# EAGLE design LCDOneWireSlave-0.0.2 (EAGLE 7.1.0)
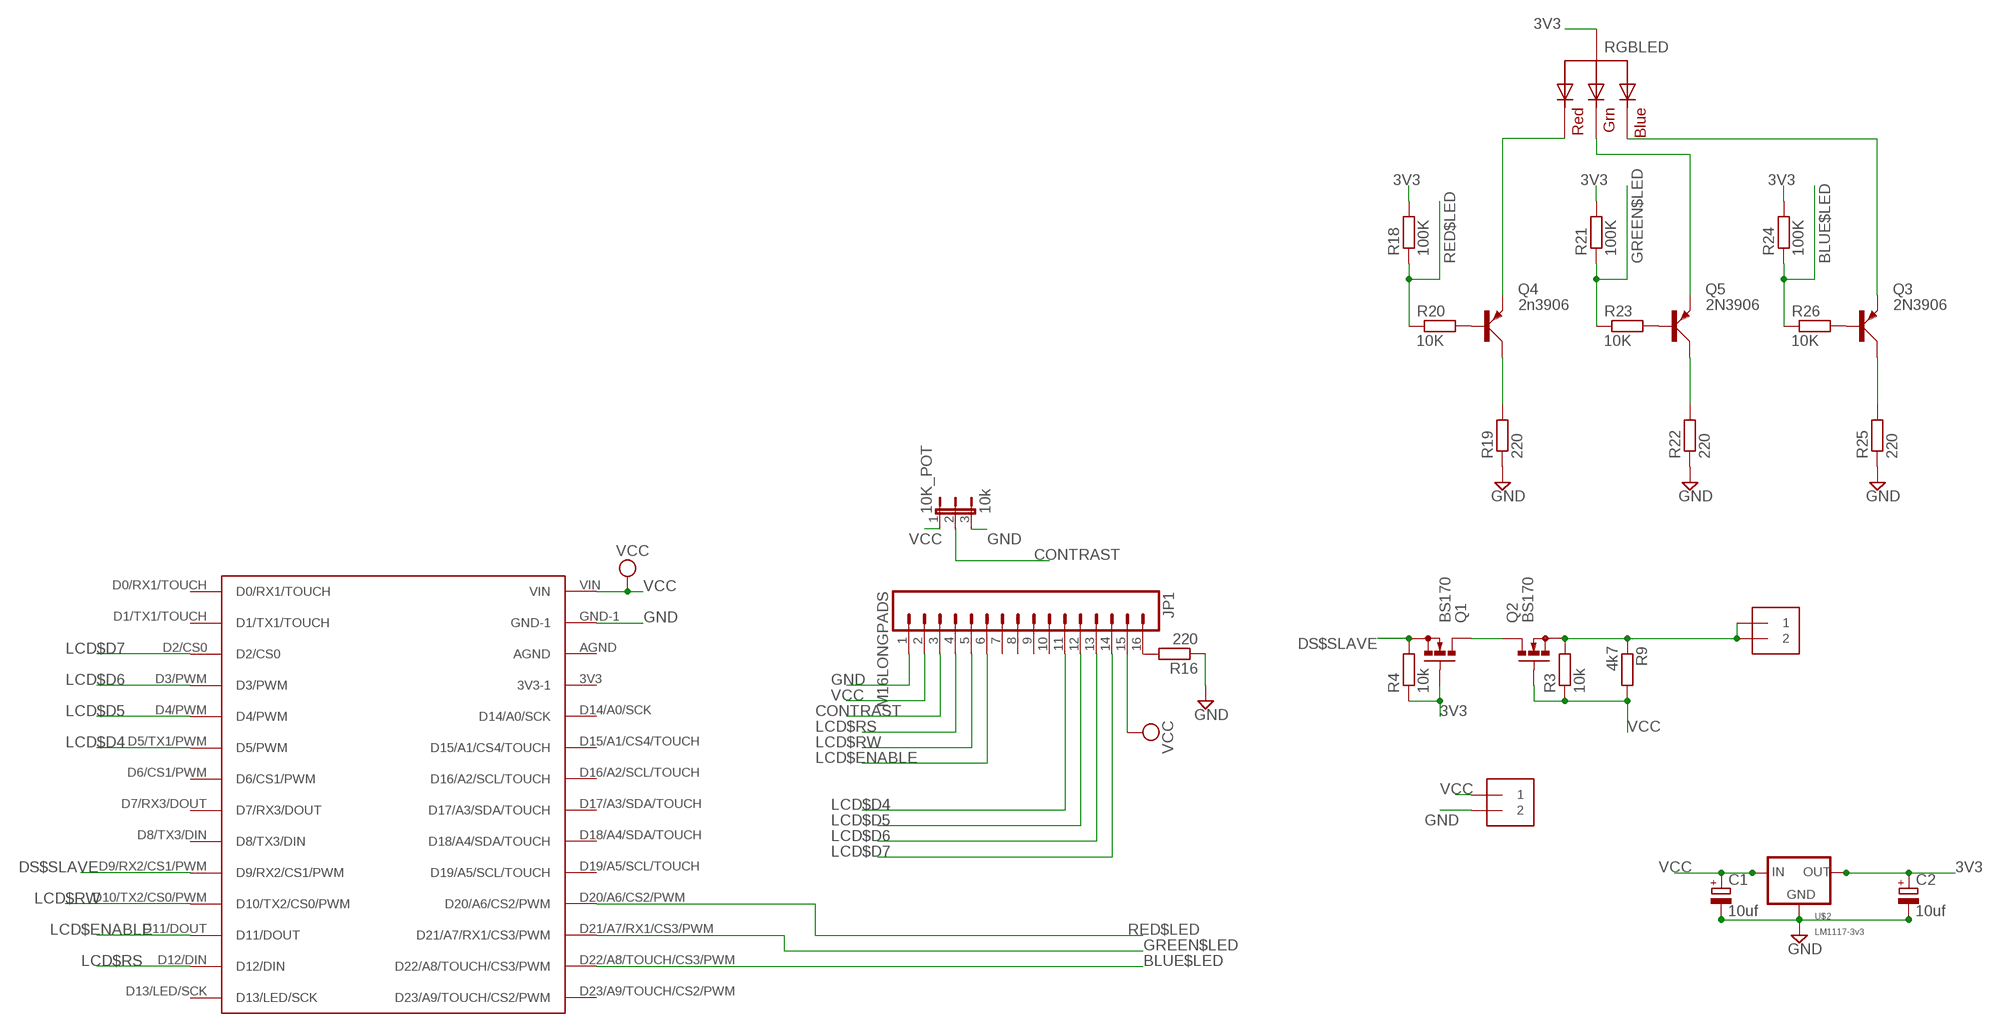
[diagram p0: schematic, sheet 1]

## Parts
10K_POT  10k  JP2E  [JP2]
C1  10uf  CPOL-EUE5-4  [E5-4]
C2  10uf  CPOL-EUE5-4  [E5-4]
DATA  1X2-3.5MM  [1X2-3.5MM]
JP1  M16LONGPADS  [1X16_LONGPADS]
POWER  1X2-3.5MM  [1X2-3.5MM]
Q1  BS170  [SOT54E]
Q2  BS170  [SOT54E]
Q3  2N3906  [TO92D]
Q4  2n3906  2N3906  [TO92D]
Q5  2N3906  [TO92D]
R3  10k  R-EU_0207/10  [0207/10]
R4  10k  R-EU_0207/10  [0207/10]
R9  4k7  R-EU_0207/10  [0207/10]
R16  220  R-EU_0207/10  [0207/10]
R18  100K  R-EU_0207/10  [0207/10]
R19  220  R-EU_0207/10  [0207/10]
R20  10K  R-EU_0207/10  [0207/10]
R21  100K  R-EU_0207/10  [0207/10]
R22  220  R-EU_0207/10  [0207/10]
R23  10K  R-EU_0207/10  [0207/10]
R24  100K  R-EU_0207/10  [0207/10]
R25  220  R-EU_0207/10  [0207/10]
R26  10K  R-EU_0207/10  [0207/10]
RGBLED  RGBLED_CA-5MM  [LED5MMRGB]
U$1  TEENSY30-FULL  [TEENSY30-FULL]
U$2  LM1117-3v3  V_REG_LD1117VXX  [78XXL]

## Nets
3V3 [3v3]: C2.+ Q1.G R4.1 R18.2 R21.2 R24.2 RGBLED.2(VCC) U$2.GND(OUT)
BLUE$LED: R24.1 R26.1 U$1.D22/A8/TOUCH/CS3/PWM
CONTRAST: 10K_POT.2 JP1.3
DS$SLAVE: Q1.S R4.2 U$1.D9/RX2/CS1/PWM
GND [GND]: 10K_POT.3 C1.- C2.- JP1.1 POWER.2 R16.1 R19.1 R22.1 R25.1 U$1.GND-1 U$2.IN(GND)
GREEN$LED: R21.1 R23.1 U$1.D21/A7/RX1/CS3/PWM
LCD$D4: JP1.11 U$1.D5/TX1/PWM(D5/PWM)
LCD$D5: JP1.12 U$1.D4/PWM
LCD$D6: JP1.13 U$1.D3/PWM
LCD$D7: JP1.14 U$1.D2/CS0
LCD$ENABLE: JP1.6 U$1.D11/DOUT
LCD$RS: JP1.4 U$1.D12/DIN
LCD$RW: JP1.5 U$1.D10/TX2/CS0/PWM
N$1: DATA.1 DATA.2 Q2.S R3.2 R9.1
N$2: Q4.E RGBLED.1(RED)
N$3: Q5.E RGBLED.3(GREEN)
N$4: Q3.E RGBLED.4(BLUE)
N$5: Q4.C R19.2
N$6: JP1.16 R16.2
N$7: Q5.C R22.2
N$8: Q3.C R25.2
N$10: Q4.B R20.2
N$15: Q5.B R23.2
N$22: Q3.B R26.2
N$26: Q1.D Q2.D
RED$LED: R18.1 R20.1 U$1.D20/A6/CS2/PWM
VCC [VCC]: 10K_POT.1 C1.+ JP1.2 JP1.15 POWER.1 Q2.G R3.1 R9.2 U$1.VIN U$2.OUT(IN)
Unconnected: JP1.7 JP1.8 JP1.9 JP1.10 U$1.3V3(3V3-1) U$1.AGND U$1.D0/RX1/TOUCH U$1.D1/TX1/TOUCH U$1.D6/CS1/PWM U$1.D7/RX3/DOUT U$1.D8/TX3/DIN U$1.D13/LED/SCK U$1.D14/A0/SCK U$1.D15/A1/CS4/TOUCH U$1.D16/A2/SCL/TOUCH U$1.D17/A3/SDA/TOUCH U$1.D18/A4/SDA/TOUCH U$1.D19/A5/SCL/TOUCH U$1.D23/A9/TOUCH/CS2/PWM

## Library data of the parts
10K_POT = jumper:JP2E: JUMPER
C1 C2 = resistor:CPOL-EU: POLARIZED CAPACITOR, European symbol
DATA POWER = Adafruit:1X2: 3.5mm Terminal block
JP1 = SparkFun-Connectors:M16: 1x16 .1" header
Q1 Q2 = BS170-inline:BS170: N-CHANNEL MOS FET
Q3-Q5 = transistor-small-signal:2N3906: PNP TRANSISTOR
R3 R4 R9 = rcl:R-EU_: RESISTOR, European symbol
R16 R18-R26 = resistor:R-EU_: RESISTOR, European symbol
RGBLED = Adafruit:RGBLED_CA: RGB LED, common-anode 5MM Staggered pins 5mm Piranha package http://www.ladyada.net/library/pcb/eaglelibrary.html
U$1 = teensy30:TEENSY30-FULL
U$2 = LM1117-TO22V:V_REG_LD1117VXX: LD1117 3V3 Regulator in TO-220 package.

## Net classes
1 VCC: width 0.508 mm
2 GND: width 0.508 mm
3 3v3: width 0.508 mm

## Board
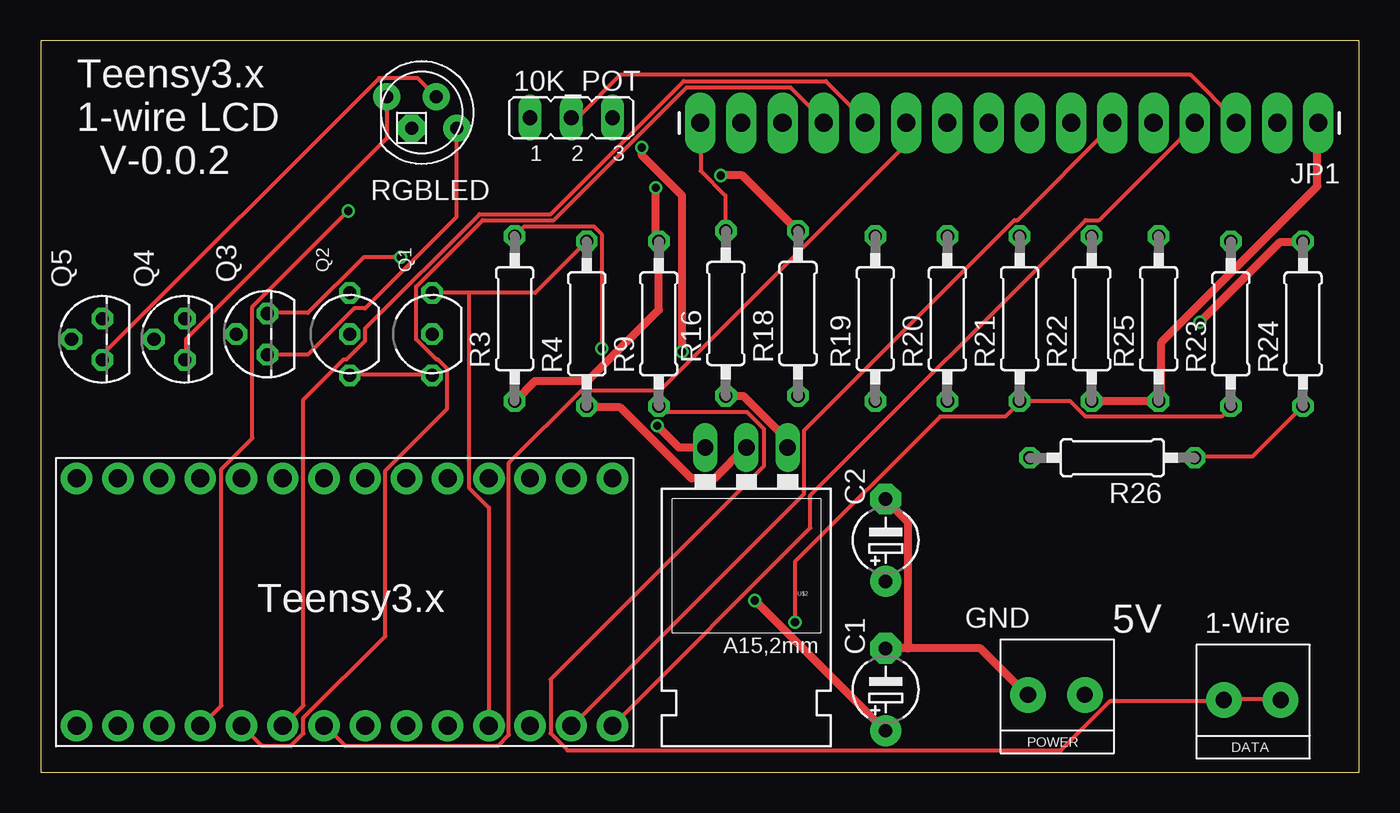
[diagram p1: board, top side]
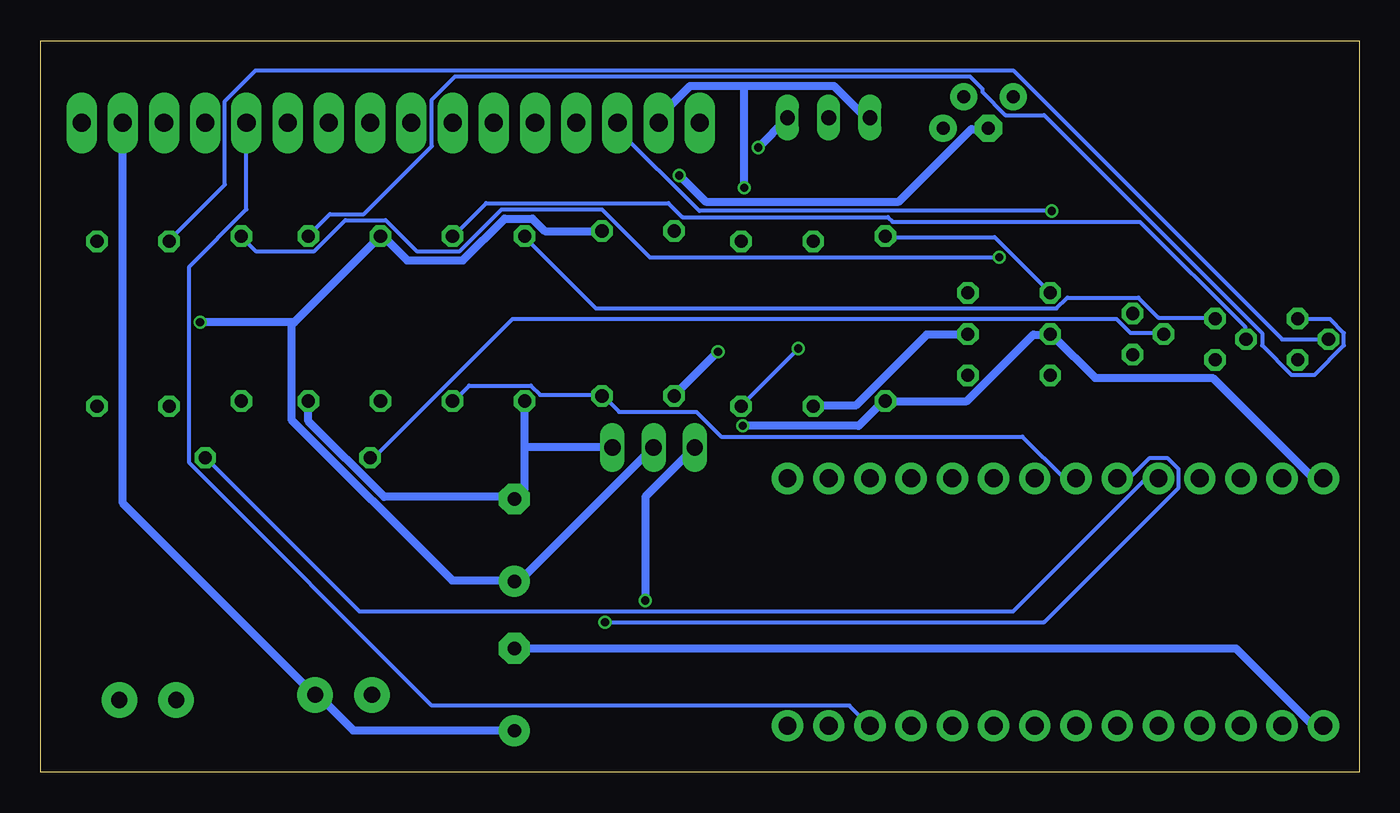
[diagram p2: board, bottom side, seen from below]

Size 81.27 x 45.08 mm. Coordinates in mm from the lower left corner, seen from the top.
Outline: 0,0 81.27,0 81.27,45.08 0,45.08 0,0
Copper layers (1*16): Top 0.035mm / dielectric 1.5mm / Bottom 0.035mm
Design rules "dirt_cheap_dirty_boards.v2.jlm.": minimum track width 10mil, minimum drill 20mil, track to track 5mil, track to pad 5mil, pad to pad 5mil, via to via 5mil, smd to smd 0mil, copper to edge 10mil, drill to drill 10mil, minimum pad ring 10mil, minimum via ring 6mil, stop-mask expansion 2mil, vias tented up to drill 25mil, thermal gap 10mil

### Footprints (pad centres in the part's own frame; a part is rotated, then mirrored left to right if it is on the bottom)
JP2 = drill 0.914 long: 1 -2.54,0; 2 0,0; 3 2.54,0
E5-4 = drill 0.813 pad 1.905: + -2.54,0 | drill 0.813 pad 1.905 octagon: - 2.54,0
1X2-3.5MM = drill 1 pad 2.184: 1 1.8,0; 2 -1.7,0
1X16_LONGPADS = drill 1.118 pad 1.88 long: 1 0,0; 2 2.54,0; 3 5.08,0; 4 7.62,0; 5 10.16,0; 6 12.7,0; 7 15.24,0; 8 17.78,0; 9 20.32,0; 10 22.86,0; 11 25.4,0; 12 27.94,0; 13 30.48,0; 14 33.02,0; 15 35.56,0; 16 38.1,0
SOT54E = drill 0.813 octagon: D -1.27,0; G 1.27,0; S 3.81,0
TO92D = drill 0.813 octagon: B 0,1.905; C 1.27,0; E -1.27,0
0207/10 = drill 0.813 octagon: 1 -5.08,0; 2 5.08,0
LED5MMRGB = drill 0.8 pad 1.676: 1 -2.159,0.968; 3 0.889,0.968; 4 2.159,-0.968 | drill 0.8 pad 1.676 octagon: 2 -0.635,-0.968
TEENSY30-FULL = drill 1.1 pad 1.93: 3V3 7.62,11.43; AGND 7.62,13.97; D0/RX1/TOUCH -7.62,13.97; D1/TX1/TOUCH -7.62,11.43; D2/CS0 -7.62,8.89; D3/PWM -7.62,6.35; D4/PWM -7.62,3.81; D5/TX1/PWM -7.62,1.27; D6/CS1/PWM -7.62,-1.27; D7/RX3/DOUT -7.62,-3.81; D8/TX3/DIN -7.62,-6.35; D9/RX2/CS1/PWM -7.62,-8.89; D10/TX2/CS0/PWM -7.62,-11.43; D11/DOUT -7.62,-13.97; D12/DIN -7.62,-16.51; D13/LED/SCK 7.62,-16.51; D14/A0/SCK 7.62,-13.97; D15/A1/CS4/TOUCH 7.62,-11.43; D16/A2/SCL/TOUCH 7.62,-8.89; D17/A3/SDA/TOUCH 7.62,-6.35; D18/A4/SDA/TOUCH 7.62,-3.81; D19/A5/SCL/TOUCH 7.62,-1.27; D20/A6/CS2/PWM 7.62,1.27; D21/A7/RX1/CS3/PWM 7.62,3.81; D22/A8/TOUCH/CS3/PWM 7.62,6.35; D23/A9/TOUCH/CS2/PWM 7.62,8.89; GND-1 -7.62,16.51; VIN 7.62,16.51
78XXL = drill 1.016 long: GND 0,-3.81; IN -2.54,-3.81; OUT 2.54,-3.81

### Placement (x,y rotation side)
10K_POT  32.7,40.32 0 top
C1  52.07,5.08 90 top
C2  52.07,14.29 90 top
DATA  74.61,4.45 0 top
JP1  78.74,40.01 180 top
POWER  62.55,4.76 0 top
Q1  24.13,25.72 90 top
Q2  19.05,25.72 90 top
Q3  13.97,26.99 90 top
Q4  8.89,26.67 90 top
Q5  3.81,26.67 90 top
R3  29.21,27.94 90 top
R4  33.66,27.62 90 top
R9  38.1,27.62 90 top
R16  42.23,28.26 90 top
R18  46.67,28.26 90 top
R19  51.44,27.94 90 top
R20  55.88,27.94 90 top
R21  60.33,27.94 90 top
R22  64.77,27.94 90 top
R23  73.34,27.62 90 top
R24  77.79,27.62 90 top
R25  68.9,27.94 90 top
R26  66.04,19.37 180 top
RGBLED  23.5,40.64 0 top
U$1  18.73,10.48 90 top
U$2  43.5,16.19 180 top

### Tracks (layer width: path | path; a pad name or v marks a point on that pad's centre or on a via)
3V3  (via drill 0.51)
  Top 0.508: R4.1 33.72,22.48 35.72,22.48 40.1,18.1 41.53,18.1 43.43,20 U$2.GND | v71.44,27.72 76.39,32.67 77.72,32.67 R24.2 | v41.91,36.77 43.24,36.77 R18.2
  Bottom 0.508: R4.1 33.62,22.57 31.05,22.57 26.67,26.96 24.19,26.96 Q1.G | U$2.GND 43.53,20 51.72,11.81 52.01,11.81 C2.+ 52.29,11.81 55.91,11.81 65.82,21.72 65.82,27.72 | 65.82,27.72 65.63,27.72 R21.2 60.1,32.96 58.67,31.53 55.24,31.53 52.67,34.1 50.96,34.1 50.2,33.34 R18.2 | 65.82,27.72 v71.44,27.72 | v41.91,36.77 40.29,35.15 28.38,35.15 23.91,39.62 22.86,39.62 RGBLED.2
BLUE$LED
  Top 0.254: R24.1 74.68,19.43 71.15,19.43 R26.1
  Bottom 0.254: U$1.D22/A8/TOUCH/CS3/PWM 13.14,18.1 21.34,9.91 61.63,9.91 71.06,19.34 R26.1
CONTRAST
  Top 0.254: 10K_POT.2 32.77,40.39 33.15,40.39 35.72,42.96 70.87,42.96 73.63,40.2 73.63,40.01 JP1.3
DS$SLAVE
  Top 0.254: 26.38,29.53 30.48,29.53 R4.2 | 26.38,29.53 Q1.S | U$1.D9/RX2/CS1/PWM 27.62,16.29 26.38,17.53 26.38,29.53
GND  (via drill 0.51)
  Top 0.508: 53.44,7.62 57.91,7.62 60.77,4.76 POWER.2 | 53.44,7.62 C1.- | R22.1 R25.1 69.06,23.05 69.06,26.48 78.68,36.1 78.68,40.01 JP1.1 | R16.1 42.29,23.15 43.34,23.15 46.01,20.48 46.01,20 U$2.IN | v37.05,38.48 37.05,38.01 39.53,35.53 v39.53,25.91 | 53.44,7.62 53.44,15.43 52.1,16.76 C2.-
  Bottom 0.508: U$1.GND-1 2.86,2.86 7.62,7.62 C1.- | 51.44,20 51.44,17.43 52.01,16.86 C2.- 52.29,16.95 60.1,16.95 64.77,21.62 R22.1 | 51.44,20 R19.1 | v37.05,38.48 35.24,40.29 10K_POT.3 | v39.53,25.91 42.2,23.24 R16.1 | U$2.IN 51.44,20
GREEN$LED  (via drill 0.51)
  Top 0.254: R23.1 73.34,22.48 72.77,21.91 64.39,21.91 63.44,22.86 R21.1 60.29,22.77 59.44,21.91 55.44,21.91 46.48,12.95 v46.48,9.24
  Bottom 0.254: U$1.D21/A7/RX1/CS3/PWM 14.19,18.1 12.95,19.34 11.81,19.34 11.14,18.67 11.14,17.53 19.43,9.24 v46.48,9.24
LCD$D4
  Top 0.254: JP1.11 53.34,38.67 38.2,23.53 33.34,23.53 28.86,19.05 28.86,2.29 28.19,1.62 18.76,1.62 17.53,2.86 U$1.D5/TX1/PWM
LCD$D5
  Top 0.254: JP1.12 50.77,40.01 50.77,40.2 48.39,42.58 39.62,42.58 31.43,34.38 27.05,34.38 20,27.34 20,26.57 18.86,25.43 18.67,25.43 16.19,22.95 16.19,4.1 14.95,2.86 U$1.D4/PWM
LCD$D6
  Top 0.254: U$1.D3/PWM 13.62,1.62 15.43,1.62 16.19,2.38 16.19,3.33 21.24,8.38 21.24,18.57 25.05,22.38 25.05,24.86 24.48,25.43 24.38,25.43 23.15,26.67 23.15,29.91 27.24,34 31.62,34 39.81,42.2 46.2,42.2 48.2,40.2 48.2,40.01 JP1.13
LCD$D7  (via drill 0.51)
  Top 0.254: v18.95,34.58 13.05,28.67 13.05,20.57 11.14,18.67 11.14,4.1 9.91,2.86 U$1.D2/CS0
  Bottom 0.254: JP1.14 45.72,39.62 40.67,34.58 v18.95,34.58
LCD$ENABLE
  Top 0.254: JP1.6 66.01,40.01 66.01,39.81 60.2,34 60.01,34 47.05,21.05 47.05,17.14 32.77,2.86 U$1.D11/DOUT
LCD$RS
  Top 0.254: U$1.D12/DIN 47.43,15.05 47.43,17.05 64.39,34 65.25,34 71.06,39.81 71.06,40.01 JP1.4
LCD$RW
  Bottom 0.254: JP1.5 68.58,34.67 72.1,31.15 72.1,19.05 57.15,4.1 31.43,4.1 30.19,2.86 U$1.D10/TX2/CS0/PWM
N$1  (via drill 0.51)
  Top 0.254: DATA.1 76.39,4.48 72.96,4.48 DATA.2 72.87,4.38 65.91,4.38 62.87,1.33 32.48,1.33 31.43,2.38 31.43,5.71 44.58,18.86 44.58,21.14 43.53,22.19 38.39,22.19 38.1,22.48 R9.1 | v34.58,26.1 34.58,33.15 34.1,33.62 29.81,33.62 R3.2
  Bottom 0.254: v34.58,26.1 38.1,22.57 R9.1 | Q2.S 22.48,32.96 29.15,32.96 R3.2
N$2
  Top 0.254: RGBLED.1 21.34,39.05 8.95,26.67 8.95,25.43 Q4.E
N$3
  Top 0.254: Q5.E 3.81,25.72 20.86,42.77 23.24,42.77 24.38,41.62 RGBLED.3
N$4
  Top 0.254: Q3.E 16.48,25.72 19.34,28.57 20,28.57 25.62,34.2 25.62,39.62 RGBLED.4
N$5
  Bottom 0.254: Q4.C 8.95,28 12.38,28 13.62,29.24 18,29.24 18.67,28.57 47.05,28.57 51.44,32.96 R19.2
N$6
  Top 0.254: R16.2 42.2,33.34 42.2,35.53 40.67,37.05 40.67,40.01 JP1.16
N$7
  Bottom 0.254: Q5.C 3.81,27.91 1.81,27.91 0.95,27.05 0.95,26.29 2.76,24.48 4.19,24.48 6,26.29 6,27.05 19.43,40.48 21.81,40.48 23.24,41.91 23.24,42.1 24,42.86 55.72,42.86 57.15,41.43 57.15,38.58 61.34,34.38 63.44,34.38 64.77,33.05 R22.2
N$8  (via drill 0.51)
  Top 0.254: v22.19,31.72 19.91,31.72 16.48,28.29 14,28.29 Q3.C
  Bottom 0.254: v22.19,31.72 43.72,31.72 46.67,34.67 52.86,34.67 55.44,32.1 58.1,32.1 60.01,34 62.48,34 64.39,32.1 68.01,32.1 68.87,32.96 R25.2
N$10
  Bottom 0.254: Q4.B 7.05,26.67 7.05,27.43 13.53,33.91 28.77,33.91 29.05,34.2 41.72,34.2 42.58,35.05 53.82,35.05 55.82,33.05 R20.2
N$15
  Bottom 0.254: Q5.B 4.76,26.67 21.34,43.24 68.01,43.24 69.91,41.34 69.91,36.2 73.34,32.77 R23.2
N$22
  Bottom 0.254: R26.2 60.96,19.43 60.67,19.43 52.2,27.91 14.95,27.91 14.1,27.05 12.1,27.05 Q3.B
N$26
  Top 0.254: Q2.D 19.05,24.48 24.1,24.48 Q1.D
RED$LED
  Bottom 0.254: R20.1 55.82,22.86 54.86,23.81 51.05,23.81 50.48,23.24 46.67,23.24 R18.1 46.58,23.15 45.62,22.19 40.86,22.19 39.34,20.67 20.77,20.67 18.19,18.1 U$1.D20/A6/CS2/PWM
VCC  (via drill 0.51)
  Top 0.508: R3.1 29.24,22.86 30.48,24.1 33.72,24.1 38.1,28.48 R9.2 37.91,32.86 v37.91,36.01 | U$2.OUT 39.34,20 v38.01,21.34 | v44.01,10.57 52.01,2.57 C1.+
  Bottom 0.508: JP1.2 76.2,16.57 64.39,4.76 POWER.1 64.1,4.67 62.01,2.57 52.1,2.57 C1.+ | 37.91,42.29 41.24,42.29 43.15,40.39 43.15,40.01 JP1.15 | 37.91,42.29 32.38,42.29 30.48,40.39 30.19,40.39 10K_POT.1 | v38.01,21.34 30.86,21.34 29.43,22.77 R3.1 24.19,22.86 20.1,26.96 19.05,26.96 Q2.G 18.86,26.86 16.29,24.29 9.05,24.29 2.86,18.1 U$1.VIN | v37.91,36.01 37.91,42.29 | v44.01,10.57 44.01,16.95 U$2.OUT

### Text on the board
tNames: Teensy3.x / 1-wire LCD / V-0.0.2 | Teensy3.x | GND | 5V | 1-Wire

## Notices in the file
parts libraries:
SparkFun-Connectors: Licensing: CC v3.0 Share-Alike You are welcome to use this library for commercial purposes.
